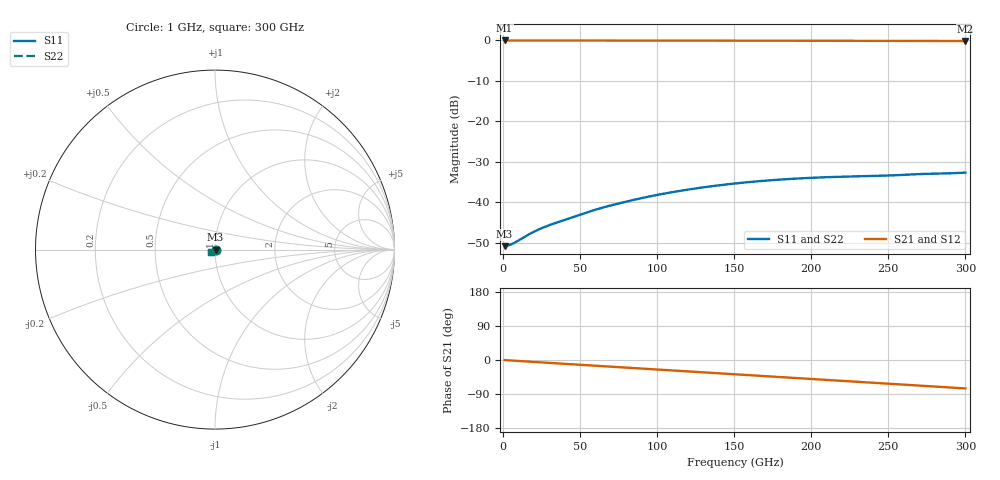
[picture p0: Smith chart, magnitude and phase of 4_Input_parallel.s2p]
#  Hz  S  RI  R  50
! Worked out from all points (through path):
!   300 points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, 1 GHz to 300 GHz, reference 50 ohm
!   highest |S21| = -0.02 dB at 1 GHz (marker M1); lowest = -0.2 dB at 300 GHz (marker M2)
!   group delay of S21, straight-line fit = 694 fs
!   lowest |S11| = -50.8 dB at 1 GHz (marker M3), VSWR 1.01, Z = 50.3 + j0.000782 ohm
!   |S11| at or under -10 dB: start of sweep to end of sweep
!   |S22| runs from -50.8 to -32.7 dB; largest |S21 - S12| = 0.00018
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1e9  0.00288 7.78e-06  0.9972 -0.00453  0.9972 -0.00453  0.00288 6.63e-06
3e9  0.00292 1.73e-05  0.997 -0.0136  0.997 -0.0136  0.00293 1.4e-05
6e9  0.00307 -4.8e-06  0.9966 -0.0271  0.9965 -0.0271  0.00307 -1.03e-05
9e9  0.00329 -9.71e-05  0.9958 -0.0405  0.9958 -0.0405  0.00329 -0.000103
1.8e10  0.00405 -0.000889  0.9925 -0.08  0.9925 -0.08  0.00404 -0.000887
2.5e10  0.00441 -0.00187  0.9892 -0.1102  0.9891 -0.1102  0.00441 -0.00187
3.2e10  0.00453 -0.00291  0.9851 -0.1404  0.9851 -0.1404  0.00454 -0.0029
5.1e10  0.00439 -0.00565  0.969 -0.2214  0.969 -0.2214  0.00439 -0.00565
6.1e10  0.00402 -0.00717  0.9581 -0.2633  0.9581 -0.2633  0.00402 -0.00717
7.2e10  0.00335 -0.00876  0.944 -0.3089  0.944 -0.3088  0.00335 -0.00876
8.7e10  0.00217 -0.0107  0.9212 -0.3696  0.9212 -0.3696  0.00217 -0.0107
1.01e11  0.00076 -0.0124  0.8966 -0.4249  0.8966 -0.4248  0.000761 -0.0124
1.13e11  -0.000643 -0.0137  0.8728 -0.4709  0.8728 -0.471  -0.000644 -0.0137
1.26e11  -0.0023 -0.0148  0.8445 -0.5194  0.8445 -0.5194  -0.0023 -0.0148
1.51e11  -0.00578 -0.0161  0.7824 -0.6077  0.7824 -0.6077  -0.00578 -0.0161
1.75e11  -0.00915 -0.0164  0.7141 -0.6857  0.7141 -0.6857  -0.00915 -0.0164
2.01e11  -0.0124 -0.0158  0.6311 -0.7615  0.6311 -0.7615  -0.0124 -0.0158
2.27e11  -0.0149 -0.0146  0.5396 -0.827  0.5396 -0.8269  -0.0149 -0.0146
2.51e11  -0.0166 -0.0136  0.4491 -0.877  0.4491 -0.877  -0.0166 -0.0136
2.76e11  -0.0188 -0.0124  0.3512 -0.9185  0.3513 -0.9185  -0.0188 -0.0124
2.9e11  -0.0197 -0.0115  0.2948 -0.9368  0.2947 -0.9368  -0.0197 -0.0115
3e11  -0.0206 -0.0109  0.2541 -0.9482  0.2542 -0.948  -0.0205 -0.0109
